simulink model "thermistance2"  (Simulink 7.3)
settings: Solver=ode14x  SolverMode=SingleTasking  StartTime=0.0  StopTime=1  FixedStep=1  MaxStep=1e-6  RelTol=1e-3
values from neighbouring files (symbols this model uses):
  R = 1e3    (= 1000)    [oscillateur_dephasage.m]    (also in Calcul_Ampl_phase_A.m = 1; circuit_RLC_parallele_.m = 4; symbolique_circuit_RC.m = 4; parametres.m = 4)
libraries: fl_lib x13, nesl_utility x4, elec_lib x2

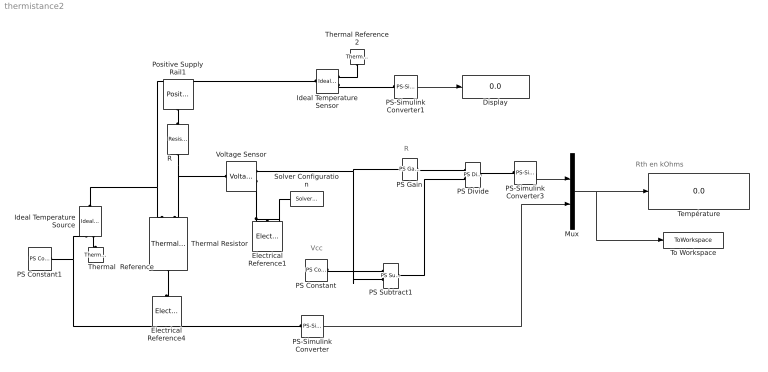
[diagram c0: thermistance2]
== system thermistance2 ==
  note: Rth en kOhms
  note: R
  note: Vcc
  Display : Display
  Electrical Reference1 : fl_lib/Electrical/Electrical Elements/Electrical Reference  DialogController=NetworkEngine.DynNeDlgSource  SystemSampleTime=-1  i_Log=off  LocalVarNames=|i  LocalVarDescs=|i  LocalVarLogging=0
  Electrical Reference4 : fl_lib/Electrical/Electrical Elements/Electrical Reference  DialogController=NetworkEngine.DynNeDlgSource  SystemSampleTime=-1  i_Log=off  LocalVarNames=|i  LocalVarDescs=|i  LocalVarLogging=0
  Ideal Temperature Sensor : fl_lib/Thermal/Thermal Sensors/Ideal Temperature Sensor  DialogController=NetworkEngine.DynNeDlgSource  SystemSampleTime=-1  Qs_Log=off  Ts_Log=off  LocalVarNames=|Qs|Ts  LocalVarDescs=|Qs|Ts  LocalVarLogging=[0 0]
  Ideal Temperature Source : fl_lib/Thermal/Thermal Sources/Ideal Temperature Source  DialogController=NetworkEngine.DynNeDlgSource  SystemSampleTime=-1  Q_Log=off  T_Log=off  LocalVarNames=|Q|T  LocalVarDescs=|Q|T  LocalVarLogging=[0 0]
  Mux : Mux  Inputs=2
  PS Constant : fl_lib/Physical Signals/Sources/PS Constant  DialogController=NetworkEngine.DynNeDlgSource  SystemSampleTime=-1  constant=Vcc  LocalVarLogging=[]
  PS Constant1 : fl_lib/Physical Signals/Sources/PS Constant  DialogController=NetworkEngine.DynNeDlgSource  SystemSampleTime=-1  constant=temp  LocalVarLogging=[]
  PS Divide : fl_lib/Physical Signals/Functions/PS Divide  DialogController=NetworkEngine.DynNeDlgSource  SystemSampleTime=-1  LocalVarLogging=[]
  PS Gain : fl_lib/Physical Signals/Functions/PS Gain  DialogController=NetworkEngine.DynNeDlgSource  SystemSampleTime=-1  gain=R  LocalVarLogging=[]
  PS Subtract1 : fl_lib/Physical Signals/Functions/PS Subtract  DialogController=NetworkEngine.DynNeDlgSource  SystemSampleTime=-1  LocalVarLogging=[]
  PS-Simulink Converter : nesl_utility/PS-Simulink Converter  DialogController=NetworkEngine.DynNeUtilDlgSource  SystemSampleTime=-1  PhysicalDomain=network_engine_domain  LeftPortType=input  RightPortType=output  SubClassName=ps_output  Unit=1  AffineConversion=off
  PS-Simulink Converter1 : nesl_utility/PS-Simulink Converter  DialogController=NetworkEngine.DynNeUtilDlgSource  SystemSampleTime=-1  PhysicalDomain=network_engine_domain  LeftPortType=input  RightPortType=output  SubClassName=ps_output  Unit=1  AffineConversion=off
  PS-Simulink Converter3 : nesl_utility/PS-Simulink Converter  DialogController=NetworkEngine.DynNeUtilDlgSource  SystemSampleTime=-1  PhysicalDomain=network_engine_domain  LeftPortType=input  RightPortType=output  SubClassName=ps_output  Unit=1  AffineConversion=off
  Positive Supply Rail1 : elec_lib/Sources/Positive Supply Rail  DialogController=NetworkEngine.DynNeDlgSource  SystemSampleTime=-1  v0=Vcc V  current_Log=off  voltage_Log=off  power_Log=off  LocalVarNames=|current|voltage|power  LocalVarDescs=|Current (A)|Voltage (V)|Power (W)  LocalVarLogging=[0 0 0]
  R : fl_lib/Electrical/Electrical Elements/Resistor  DialogController=NetworkEngine.DynNeDlgSource  SystemSampleTime=-1  R=R kOhm  i_Log=off  v_Log=off  LocalVarNames=|i|v  LocalVarDescs=|i|v  LocalVarLogging=[0 0]
  Solver Configuration : nesl_utility/Solver Configuration  DialogController=NetworkEngine.DynNeUtilDlgSource  SystemSampleTime=-1  PhysicalDomain=network_engine_domain  LeftPortType=input  RightPortType=generic  SubClassName=solver  Accelerate=off  Profile=off  ResidualTolerance=1e-9  MaxNonlinIter=12  MaxModeIter=2  DoFixedCost=off  DoDC=on  LinearAlgebra=Full
  Température : Display
  Thermal  Reference : fl_lib/Thermal/Thermal Elements/Thermal Reference  DialogController=NetworkEngine.DynNeDlgSource  SystemSampleTime=-1  Q_Log=off  LocalVarNames=|Q  LocalVarDescs=|Q  LocalVarLogging=0
  Thermal Reference2 : fl_lib/Thermal/Thermal Elements/Thermal Reference  DialogController=NetworkEngine.DynNeDlgSource  SystemSampleTime=-1  Q_Log=off  LocalVarNames=|Q  LocalVarDescs=|Q  LocalVarLogging=0
  Thermal Resistor : elec_lib/Passive Devices/Thermal Resistor  DialogController=NetworkEngine.DynNeDlgSource  SystemSampleTime=-1  R0=47 kOhm  T0=25 C  alpha=5e-05 1/K  tc=10 s  K_d=0.001 W/K  init_temp=25 C  current_Log=off  voltage_Log=off  power_Log=off  temperature_Log=off  heat_flow_Log=off  LocalVarNames=|current|voltage|power|temperature|heat_flow  LocalVarDescs=|Resistor current (A)|Voltage across resistor (V)|Power (W)|Themistor temperature (K)|Heat flow (J/s)  LocalVarLogging=[0 0 0 0 0]
  To Workspace : ToWorkspace  VariableName=RT  SampleTime=-1  SaveFormat=Array
  Voltage Sensor : fl_lib/Electrical/Electrical Sensors/Voltage Sensor  DialogController=NetworkEngine.DynNeDlgSource  SystemSampleTime=-1  i1_Log=off  v1_Log=off  LocalVarNames=|i1|v1  LocalVarDescs=|i1|v1  LocalVarLogging=[0 0]
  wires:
  PS-Simulink Converter3/1 -> Mux/1
  PS-Simulink Converter/1 -> Mux/2
  Mux/1 -> To Workspace/1, Température/1
  PS-Simulink Converter1/1 -> Display/1
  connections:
  Ideal Temperature Source/LConn1 -- Thermal Resistor/LConn1 -- Ideal Temperature Sensor/LConn1
  R/LConn1 -- Thermal Resistor/LConn2 -- Voltage Sensor/LConn1
  Positive Supply Rail1/RConn1 -- R/RConn1
  Voltage Sensor/RConn2 -- Electrical Reference1/LConn1 -- Solver Configuration/RConn1
  Ideal Temperature Source/RConn2 -- Thermal  Reference/LConn1
  Thermal Resistor/RConn1 -- Electrical Reference4/LConn1
  PS Gain/RConn1 -- PS Divide/LConn1
  PS Constant/RConn1 -- PS Subtract1/LConn1
  Voltage Sensor/RConn1 -- PS Subtract1/LConn2 -- PS Gain/LConn1
  PS Subtract1/RConn1 -- PS Divide/LConn2
  PS Divide/RConn1 -- PS-Simulink Converter3/LConn1
  PS Constant1/RConn1 -- Ideal Temperature Source/RConn1 -- PS-Simulink Converter/LConn1
  Thermal Reference2/LConn1 -- Ideal Temperature Sensor/RConn1
  Ideal Temperature Sensor/RConn2 -- PS-Simulink Converter1/LConn1
